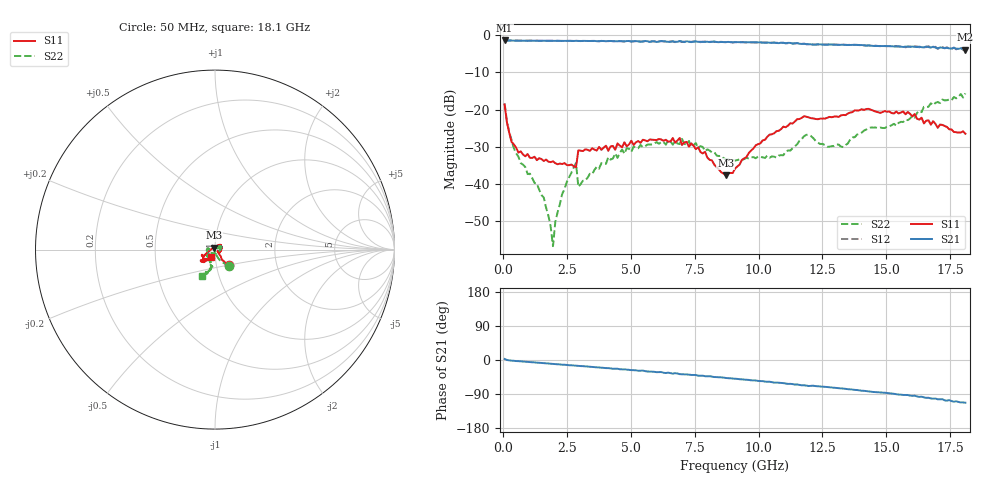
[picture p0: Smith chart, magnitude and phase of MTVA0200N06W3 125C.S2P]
! Network Analyzer HP8720D.06.14 Serial No. US36140669
! 19 Aug 2005  14:36:47
! Frequency  S11  S21  S12  S22
# HZ  S  DB R 50
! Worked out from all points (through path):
!   201 points, 50 MHz to 18.1 GHz, reference 50 ohm
!   highest |S21| = -1.41 dB at 50 MHz (marker M1); lowest = -3.9 dB at 18.1 GHz (marker M2)
!   group delay of S21, straight-line fit = 16.9 ps
!   lowest |S11| = -37.7 dB at 8.714 GHz (marker M3), VSWR 1.03, Z = 49.4 + j1.14 ohm
!   |S11| at or under -10 dB: start of sweep to end of sweep
!   |S22| runs from -56.7 to -15.7 dB; largest |S21 - S12| = 0.031
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5e7  -18.65 -48.8  -1.41 2.7  -1.41 2.5  -18.36 -50.0
3.2075e8  -28.68 -48.8  -1.42 -1.5  -1.43 -1.5  -28.13 -72.8
5.915e8  -31.56 -41.5  -1.45 -3.0  -1.47 -3.0  -32.71 -78.5
1.58425e9  -33.82 -31.1  -1.49 -8.5  -1.50 -8.4  -43.69 -105.5
1.855e9  -34.14 -30.9  -1.51 -9.9  -1.51 -9.9  -51.52 -150.2
1.94525e9  -33.94 -27.8  -1.53 -10.2  -1.51 -10.3  -56.75 167.4
2.0355e9  -34.42 -29.9  -1.52 -10.8  -1.52 -10.8  -50.32 131.1
2.48675e9  -34.93 -29.7  -1.54 -13.1  -1.53 -13.1  -39.48 81.9
2.84775e9  -35.50 -33.5  -1.50 -15.2  -1.53 -15.1  -34.39 72.9
2.938e9  -30.99 -43.1  -1.55 -15.6  -1.53 -15.6  -40.75 6.2
3.1185e9  -31.15 -38.1  -1.52 -16.2  -1.55 -16.4  -39.14 14.4
4.65275e9  -30.14 -1.1  -1.62 -24.8  -1.61 -24.9  -30.75 39.4
6.09675e9  -27.91 26.5  -1.71 -31.9  -1.62 -31.9  -29.23 29.0
7.36025e9  -29.06 40.7  -1.86 -39.5  -1.74 -39.5  -30.07 19.9
8.714e9  -37.67 118.0  -1.86 -47.4  -1.87 -47.1  -33.35 -29.9
9.075e9  -35.92 154.2  -1.85 -49.3  -1.85 -49.3  -33.72 -47.7
1.042875e10  -26.75 -159.2  -2.03 -57.3  -2.00 -58.0  -32.96 -106.2
1.21435e10  -22.38 -156.0  -2.51 -68.0  -2.49 -68.2  -27.70 171.3
1.331675e10  -21.45 -138.8  -2.55 -75.3  -2.56 -75.6  -30.07 -163.8
1.43095e10  -19.80 -140.8  -2.76 -82.9  -2.73 -83.0  -24.96 -142.4
1.512175e10  -20.54 -137.8  -2.95 -88.1  -2.90 -87.9  -24.55 -128.8
1.81e10  -26.50 -119.9  -3.89 -112.7  -3.81 -113.5  -15.66 -117.0
